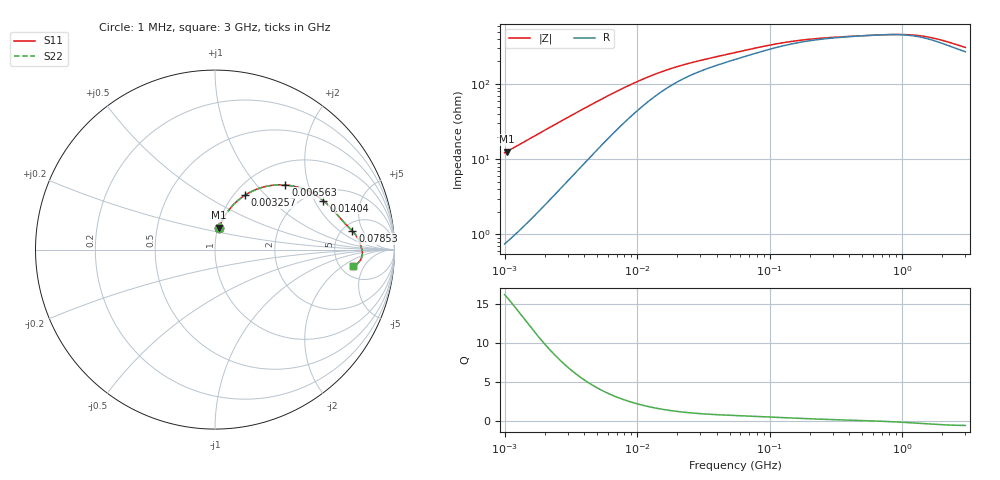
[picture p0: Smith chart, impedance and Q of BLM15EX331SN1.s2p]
! BLM15EX331SN1
# Hz S RI R 50
!Freq.(Hz) S11(Real) S11(Imag) S21(Real) S21(Imag) S12(Real) S12(Imag) S22(Real) S22(Imag)
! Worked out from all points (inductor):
!   401 points, 1 MHz to 3 GHz, reference 50 ohm
!   read as one part in series: L = 1.93 uH near 1.041 MHz
!   highest Q = 15.9 at 1.041 MHz (marker M1), where L = 1.93 uH
!   self-resonance near 677.3 MHz
!   S11 on the Smith chart (normalised r, x): 1 MHz: 1.01, +0.24; 3.257 MHz: 1.12, +0.77; 6.563 MHz: 1.44, +1.44; 14.04 MHz: 2.43, +2.36; 78.53 MHz: 6.14, +3.17; 3 GHz: 6.39, -2.95
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1000000  0.0216 0.1178  0.9784 -0.1178  0.9784 -0.1178  0.0216 0.1178
1040844  0.0232 0.1224  0.9768 -0.1224  0.9768 -0.1224  0.0232 0.1224
1462727  0.0428 0.1671  0.9572 -0.1671  0.9572 -0.1671  0.0428 0.1671
1935809  0.0707 0.2119  0.9293 -0.2119  0.9293 -0.2119  0.0707 0.2119
2511129  0.1104 0.2579  0.8896 -0.2579  0.8896 -0.2579  0.1104 0.2579
3257432  0.1672 0.3032  0.8328 -0.3032  0.8328 -0.3032  0.1672 0.3032
3823119  0.2111 0.3273  0.7889 -0.3273  0.7889 -0.3273  0.2111 0.3273
5059610  0.3014 0.3555  0.6986 -0.3555  0.6986 -0.3555  0.3014 0.3555
6563319  0.3926 0.3598  0.6074 -0.3598  0.6074 -0.3598  0.3926 0.3598
9794439  0.5204 0.3258  0.4796 -0.3258  0.4796 -0.3258  0.5204 0.3258
1.404268e7  0.6041 0.2727  0.3959 -0.2727  0.3959 -0.2727  0.6041 0.2727
1.461624e7  0.6114 0.2666  0.3886 -0.2666  0.3886 -0.2666  0.6114 0.2666
2.41077e7  0.6781 0.1975  0.3219 -0.1975  0.3219 -0.1975  0.6781 0.1975
5.477226e7  0.7427 0.1273  0.2573 -0.1273  0.2573 -0.1273  0.7427 0.1273
7.852918e7  0.766 0.1037  0.234 -0.1037  0.234 -0.1037  0.766 0.1037
1.321429e8  0.7908 0.071  0.2092 -0.071  0.2092 -0.071  0.7908 0.071
2.094008e8  0.8032 0.0463  0.1968 -0.0463  0.1968 -0.0463  0.8032 0.0463
8.005644e8  0.8201 -0.00772  0.1799 0.00772  0.1799 0.00772  0.8201 -0.00772
1.10276e9  0.8208 -0.026  0.1792 0.026  0.1792 0.026  0.8208 -0.026
1.45942e9  0.8163 -0.0459  0.1837 0.0459  0.1837 0.0459  0.8163 -0.0459
1.893158e9  0.805 -0.0658  0.195 0.0658  0.195 0.0658  0.805 -0.0658
3e9  0.7665 -0.0933  0.2335 0.0933  0.2335 0.0933  0.7665 -0.0933
